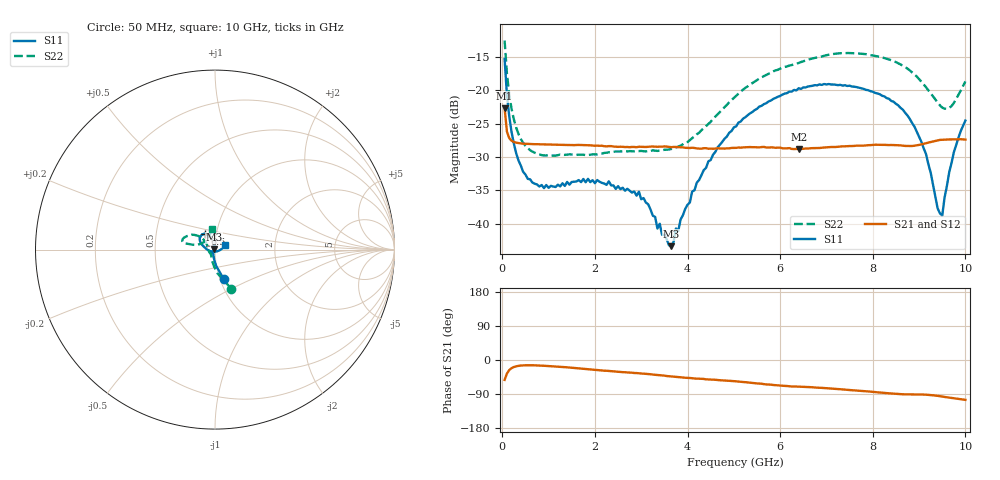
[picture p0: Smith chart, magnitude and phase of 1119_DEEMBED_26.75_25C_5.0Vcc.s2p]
!Hittite Microwave Corp.
!Digital Attenuator/PhaseShifter Rev 1.4.0
!Filename: C:\DATA\DATA\1119_DEEMBED_26.75_25C_5.0Vcc.s2p
!VNA ID: Agilent Technologies,N5224A,MY51441122,A.10.45.03
!Device type:
!2 Port Calibration.
!Temp(C): 25
!Lot Number:
!Serial Number:
!Operator:
!Misc:
!Attenuator:  26.750
# GHZ S DB R 50.0
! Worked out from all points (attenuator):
!   200 points, 50 MHz to 10 GHz, reference 50 ohm
!   highest |S21| = -22.70 dB at 50 MHz (marker M1); lowest = -28.8 dB at 6.4 GHz (marker M2)
!   lowest |S11| = -43.3 dB at 3.65 GHz (marker M3), VSWR 1.01, Z = 49.4 + j0.265 ohm
!   |S11| at or under -10 dB: start of sweep to end of sweep
!   |S22| runs from -29.8 to -12.6 dB; largest |S21 - S12| = 0.00013
!   S11 on the Smith chart (normalised r, x): 50 MHz: 1.04, -0.35; 6.5 GHz: 0.88, +0.16; 10 GHz: 1.11, +0.06
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0.05  -15.34 -73.5  -22.70 -52.4  -22.71 -52.5  -12.56 -67.3
0.1  -20.71 -85.6  -26.20 -35.9  -26.21 -35.9  -17.51 -83.9
0.2  -26.26 -97.3  -27.56 -21.6  -27.55 -21.5  -22.79 -100.5
0.45  -32.22 -113.4  -28.00 -14.2  -28.00 -14.2  -27.87 -121.3
0.9  -34.65 -129.6  -28.11 -15.2  -28.11 -15.2  -29.76 -135.8
1.75  -33.29 -136.2  -28.22 -23.1  -28.23 -23.1  -29.66 -140.7
2.95  -35.18 -128.2  -28.46 -34.9  -28.47 -35.0  -29.11 -160.0
3.35  -40.70 -143.2  -28.47 -39.6  -28.47 -39.6  -29.09 -172.1
3.4  -39.98 -153.4  -28.45 -40.0  -28.46 -40.0  -29.03 -173.6
3.65  -43.34 156.8  -28.53 -43.0  -28.53 -43.1  -28.80 177.4
4.2  -33.84 102.6  -28.71 -49.1  -28.72 -49.2  -26.60 154.0
5.05  -25.40 102.5  -28.63 -56.3  -28.64 -56.4  -20.83 138.8
6.4  -19.71 121.2  -28.83 -70.2  -28.84 -70.3  -15.93 149.9
6.5  -19.59 122.9  -28.78 -70.5  -28.80 -70.6  -15.67 151.5
6.7  -19.34 126.5  -28.67 -72.2  -28.68 -72.1  -15.25 153.9
8.35  -21.29 155.2  -28.21 -87.8  -28.21 -87.7  -15.40 168.1
8.999999  -26.92 178.5  -28.19 -90.8  -28.19 -90.9  -18.34 167.4
9.15  -29.56 -168.9  -27.94 -91.5  -27.96 -91.5  -19.56 165.4
9.400001  -37.67 -116.4  -27.51 -94.5  -27.53 -94.5  -21.84 153.7
9.5  -38.76 -58.5  -27.42 -96.6  -27.43 -96.6  -22.61 144.0
9.75  -29.30 4.1  -27.36 -100.8  -27.36 -100.8  -21.92 114.3
10  -24.55 25.5  -27.39 -105.2  -27.40 -105.2  -18.68 98.5
